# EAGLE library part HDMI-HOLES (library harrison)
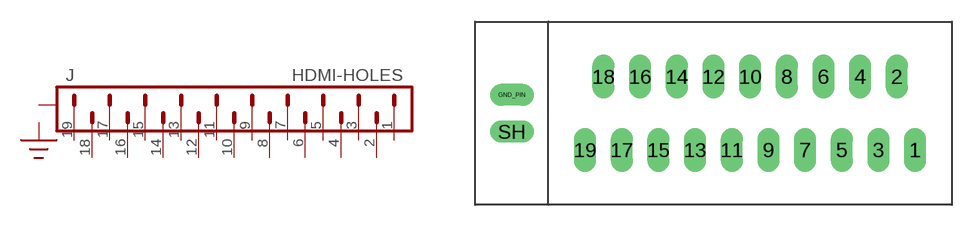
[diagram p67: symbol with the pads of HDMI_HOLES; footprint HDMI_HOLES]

Designator prefix J

## HDMI-HOLES  [HDMI_HOLES]
1  1  pas
2  2  pas
3  3  pas
4  4  pas
5  5  pas
6  6  pas
7  7  pas
8  8  pas
9  9  pas
10  10  pas
11  11  pas
12  12  pas
13  13  pas
14  14  pas
15  15  pas
16  16  pas
17  17  pas
18  18  pas
19  19  pas
GND_PIN  GND_PIN  pas
SH  SH  pas

## Footprint HDMI_HOLES (pad centres in mm)
drill 1.016 long: 1 11.43,-2.54; 2 10.16,2.54; 3 8.89,-2.54; 4 7.62,2.54; 5 6.35,-2.54; 6 5.08,2.54; 7 3.81,-2.54; 8 2.54,2.54; 9 1.27,-2.54; 10 0,2.54; 11 -1.27,-2.54; 12 -2.54,2.54; 13 -3.81,-2.54; 14 -5.08,2.54; 15 -6.35,-2.54; 16 -7.62,2.54; 17 -8.89,-2.54; 18 -10.16,2.54; 19 -11.43,-2.54; GND_PIN -16.51,1.27; SH -16.51,-1.27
